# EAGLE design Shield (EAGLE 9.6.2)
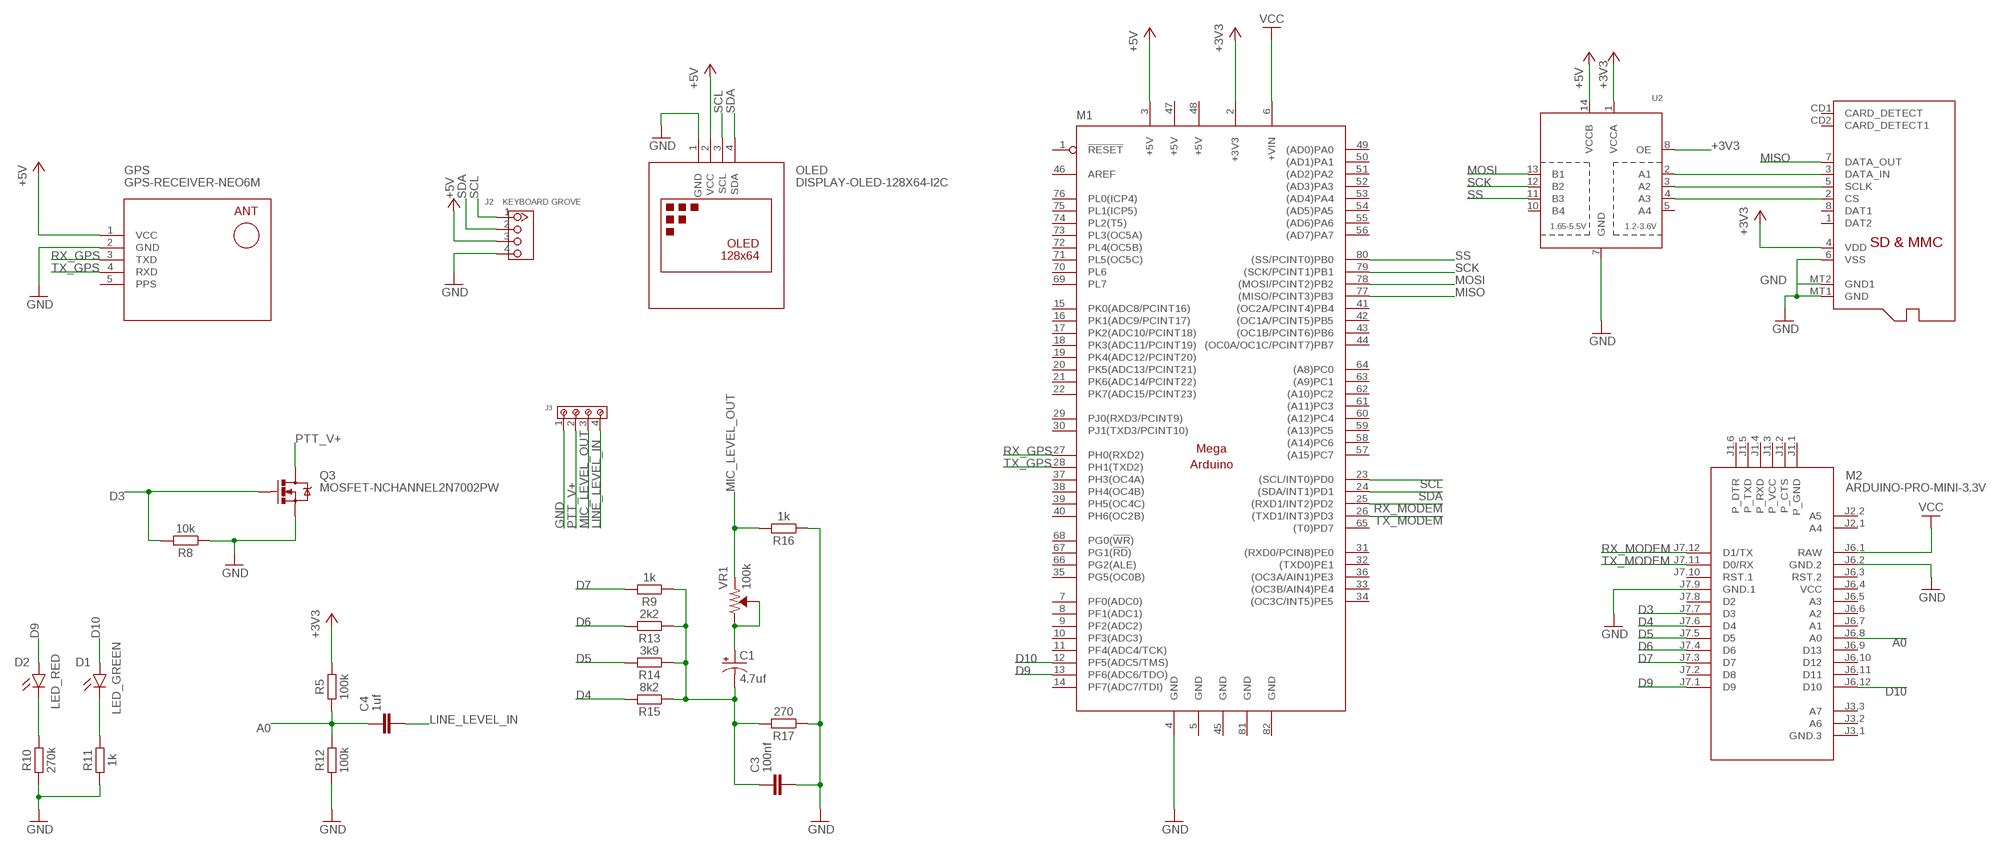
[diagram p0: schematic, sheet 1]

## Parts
C1  4.7uf  CPOL-USCT3528  [CT3528]
C3  100nf  C_CHIP-0805(2012-METRIC)  [CAPC2012X110]
C4  1uf  C_CHIP-0805(2012-METRIC)  [CAPC2012X110]
D1  LED_GREEN  CHIP-ROUND-R_0805  [LEDC2012X105N_RND-R]
D2  LED_RED  CHIP-ROUND-R_0805  [LEDC2012X105N_RND-R]
GPS  GPS-RECEIVER-NEO6M  [GPS-RECEIVER-NEO6M]
J2  KEYBOARD GROVE  GROVE-CONNECTOR-DIP-90D(4P-2.0)  [HW4-2.0-90D]
J3  691210910004  [691210910004]
M1  MEGAARDUINO_1  [MEGA_ARDUINO]
M2  ARDUINO-PRO-MINI-3.3V  [ARDUINO-PRO-MINI]
OLED  DISPLAY-OLED-128X64-I2C  [DISPLAY-OLED-128X64-I2C]
Q3  MOSFET-NCHANNEL2N7002PW  [SOT323]
R5  100k  R_CHIP-0805(2012-METRIC)  [RESC2012X65]
R8  10k  R_CHIP-0805(2012-METRIC)  [RESC2012X65]
R9  1k  R_CHIP-0805(2012-METRIC)  [RESC2012X65]
R10  270k  R_CHIP-0805(2012-METRIC)  [RESC2012X65]
R11  1k  R_CHIP-0805(2012-METRIC)  [RESC2012X65]
R12  100k  R_CHIP-0805(2012-METRIC)  [RESC2012X65]
R13  2k2  R_CHIP-0805(2012-METRIC)  [RESC2012X65]
R14  3k9  R_CHIP-0805(2012-METRIC)  [RESC2012X65]
R15  8k2  R_CHIP-0805(2012-METRIC)  [RESC2012X65]
R16  1k  R_CHIP-0805(2012-METRIC)  [RESC2012X65]
R17  270  R_CHIP-0805(2012-METRIC)  [RESC2012X65]
SD  MICROSD  [MICROSD]
U2  TXB0104PWR  [TSSOP14]
VR1  100k  TRIMPOT-SMD-3MM-CLOSED-1/8W-20%  [TRIMPOT-SMD-3MM-CLOSED]

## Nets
+3V3: M1.2(+3V3) R5.2 SD.4(VDD) U2.1(VCCA) U2.8(OE)
+5V: GPS.1(VCC) J2.3 M1.3(+5V) OLED.2(VCC) U2.14(VCCB)
A0: C4.1 M2.J6.8(A0) R5.1 R12.2
D3: M2.J7.7(D3) Q3.1(G) R8.2
D4: M2.J7.6(D4) R15.2
D5: M2.J7.5(D5) R14.2
D6: M2.J7.4(D6) R13.2
D7: M2.J7.3(D7) R9.2
D9: D2.A M1.13(PF6(ADC6/TDO)) M2.J7.1(D9)
D10: D1.A M1.12(PF5(ADC5/TMS)) M2.J6.12(D10)
GND: C3.2 GPS.2(GND) J2.4 J3.1 M1.4(GND) M2.J6.2(GND.2) M2.J7.9(GND.1) OLED.1(GND) Q3.2(S) R8.1 R10.1 R11.1 R12.1 R16.1 R17.1 SD.6(VSS) SD.MT1(GND) SD.MT2(GND1) U2.7(GND)
LINE_LEVEL_IN: C4.2 J3.4
LINE_LEVEL_OUT: C1.+ VR1.2(WIPER) VR1.3(CW)
MIC_LEVEL_OUT: J3.3 R16.2 VR1.1(CCW)
MISO: M1.77((MISO/PCINT3)PB3) SD.7(DATA_OUT)
MOSI: M1.78((MOSI/PCINT2)PB2) U2.13(B1)
N$1: SD.3(DATA_IN) U2.2(A1)
N$2: C1.- C3.1 R9.1 R13.1 R14.1 R15.1 R17.2
N$3: D2.C R10.2
N$4: D1.C R11.2
N$5: SD.5(SCLK) U2.3(A2)
N$6: SD.2(CS) U2.4(A3)
PTT_V+: J3.2 Q3.3(D)
RX_GPS: GPS.3(TXD) M1.27(PH0(RXD2))
RX_MODEM: M1.25((RXD1/INT2)PD2) M2.J7.12(D1/TX)
SCK: M1.79((SCK/PCINT1)PB1) U2.12(B2)
SCL: J2.1 M1.23((SCL/INT0)PD0) OLED.3(SCL)
SDA: J2.2 M1.24((SDA/INT1)PD1) OLED.4(SDA)
SS: M1.80((SS/PCINT0)PB0) U2.11(B3)
TX_GPS: GPS.4(RXD) M1.28(PH1(TXD2))
TX_MODEM: M1.26((TXD1/INT3)PD3) M2.J7.11(D0/RX)
VCC: M1.6(+VIN) M2.J6.1(RAW)
Unconnected: M1.1(!RESET) M1.7(PF0(ADC0)) M1.8(PF1(ADC1)) M1.9(PF2(ADC2)) M1.10(PF3(ADC3)) M1.11(PF4(ADC4/TCK)) M1.14(PF7(ADC7/TDI)) M1.15(PK0(ADC8/PCINT16)) M1.16(PK1(ADC9/PCINT17)) M1.17(PK2(ADC10/PCINT18)) M1.18(PK3(ADC11/PCINT19)) M1.19(PK4(ADC12/PCINT20)) M1.20(PK5(ADC13/PCINT21)) M1.21(PK6(ADC14/PCINT22)) M1.22(PK7(ADC15/PCINT23)) M1.29(PJ0(RXD3/PCINT9)) M1.30(PJ1(TXD3/PCINT10)) M1.31((RXD0/PCIN8)PE0) M1.32((TXD0)PE1) M1.33((OC3B/AIN4)PE4) M1.34((OC3C/INT5)PE5) M1.35(PG5(OC0B)) M1.36((OC3A/AIN1)PE3) M1.37(PH3(OC4A)) M1.38(PH4(OC4B)) M1.39(PH5(OC4C)) M1.40(PH6(OC2B)) M1.41((OC2A/PCINT4)PB4) M1.42((OC1A/PCINT5)PB5) M1.43((OC1B/PCINT6)PB6) M1.44((OC0A/OC1C/PCINT7)PB7) M1.46(AREF) M1.49((AD0)PA0) M1.50((AD1)PA1) M1.51((AD2)PA2) M1.52((AD3)PA3) M1.53((AD4)PA4) M1.54((AD5)PA5) M1.55((AD6)PA6) M1.56((AD7)PA7) M1.57((A15)PC7) M1.58((A14)PC6) M1.59((A13)PC5) M1.60((A12)PC4) M1.61((A11)PC3) M1.62((A10)PC2) M1.63((A9)PC1) M1.64((A8)PC0) M1.65((T0)PD7) M1.66(PG2(ALE)) M1.67(PG1(!RD!)) M1.68(PG0(!WR!)) M1.69(PL7) M1.70(PL6) M1.71(PL5(OC5C)) M1.72(PL4(OC5B)) M1.73(PL3(OC5A)) M1.74(PL2(T5)) M1.75(PL1(ICP5)) M1.76(PL0(ICP4)) M2.J1.1(P_GND) M2.J1.2(P_CTS) M2.J1.3(P_VCC) M2.J1.4(P_RXD) M2.J1.5(P_TXD) M2.J1.6(P_DTR) M2.J2.1(A4) M2.J2.2(A5) M2.J3.1(GND.3) M2.J3.2(A6) M2.J3.3(A7) M2.J6.3(RST.2) M2.J6.5(A3) M2.J6.6(A2) M2.J6.7(A1) M2.J6.9(D13) M2.J6.10(D12) M2.J6.11(D11) M2.J7.2(D8) M2.J7.8(D2) M2.J7.10(RST.1) SD.1(DAT2) SD.8(DAT1) SD.CD1(CARD_DETECT) SD.CD2(CARD_DETECT1) U2.5(A4) U2.10(B4)

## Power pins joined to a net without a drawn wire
+5V: M1.47(+5V) M1.48(+5V)
GND: M1.5(GND) M1.45(GND) M1.81(GND) M1.82(GND)
PPS: GPS.5(PPS)
VCC: M2.J6.4(VCC)

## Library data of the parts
C1 = adafruit:CPOL-US: POLARIZED CAPACITOR, American symbol
C3 C4 = Capacitor:C: Capacitor - Generic; CATEGORY: Capacitor
D1 = LED:CHIP-ROUND-R: LED - Generic; CATEGORY: LED; COLOR: RED; DESCRIPTION: CHIP LED ROUND; SUB-CATEGORY: CHIP; TYPE: ROUND_TOP; VALUE: LED_RED
D2 = LED:CHIP-ROUND-R: LED - Generic; CATEGORY: LED; COLOR: RED; DESCRIPTION: CHIP LED ROUND; SUB-CATEGORY: CHIP; TYPE: ROUND_TOP
GPS = diy-modules:GPS-RECEIVER-NEO6M: GPS Receiver Module based on NEO-6 device Short tutorial how to use NEO-6 module with Arduino: http://www.xarg.org/2016/06/neo6mv2-gps-module-with-arduino/ NEO-6 datasheet is available here: https://www.u-blox.com/sites/default/files/products/documents/NEO-6_DataSheet_%28GPS.G6-HW-09005%29.pdf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
J2 = OPL_Connector:GROVE-CONNECTOR-DIP-90D(4P-2.0): 320110034; VALUE: 4P-2.0-90D
J3 = Wurth_Connectors_WR-TBL Rising Cage Clamp:691210910004: WR-TBL Serie 2109 - 2.54 mm Horiz. Entry KIND PROPERTIES Pitch 2.54 mm MATERIAL PROPERTIES Insulator Material PA66 Insulator Flammability Rating UL94 V-0 Insulator Color Green Contact Material Brass Contact Plating Copper over Zinc Terminal Screw Material Steel Terminal Screw Plating Zinc Wire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; DATASHEET-URL: https://www.we-online.com/catalog/datasheet/691210910004.pdf; IR-UL: 6A; MOUNT: THT; PART-NUMBER: 691210910004; PINS: 4; PITCH: 2.54mm; TYPE: Horizontal; WIRE: 30 to 18 (AWG) 0.0509 to 0.823 (mm²); WORKING-VOLTAGE-UL: 150V (AC)
M1 = arduino:MEGAARDUINO_1: The Arduino Mega is a microcontroller board based on the ATmega1280. - 54 digital input/output pins (of which 14 can be used as PWM outputs) - 16 analog inputs - 4 UARTs (hardware serial ports) - 16 MHz crystal oscillator - USB connection - power jack - ICSP header - reset button It contains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
M2 = diy-modules:ARDUINO-PRO-MINI-*: Arduino Pro Mini and compatible devices More details available here: https://www.arduino.cc/en/Main/ArduinoBoardProMini Click here to find device on ebay.com
OLED = diy-modules:DISPLAY-OLED-128X64-I2C: 128x64 Dot Matrix OLED Module based on SSD1306 chip Variant with I2C interface More details available here: http://www.instructables.com/id/Monochrome-096-i2c-OLED-display-with-arduino-SSD13/ SSD1306 datasheet: https://cdn-shop.adafruit.com/datasheets/SSD1306.pdf Click here to find device on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
Q3 = BeagleBone_Blue_R3:MOSFET-NCHANNEL: Common NMOSFET Parts MFG P/NStore IDProd ID FDD8780TRANS-09984 SI7820DNTRANS-11055 FDS6630AIC-08089 2N7002PWTRANS-11151 FQP30N06L COM-10213TRANS-10060 BSS123LT1GTRANS-08345 BSS138TRANS-00830 BS170 2N7000; PROD_ID: TRANS-11151
R5 R8-R17 = Resistor:R: Resistor Fixed - Generic; CATEGORY: Resistor; SUB-CATEGORY: Fixed
SD = adafruit:MICROSD: Micro-SD / Transflash card holder with SPI pinout For the 3M # 2908-05WB-MG and/or 4UCON #19656 push-push type
U2 = adafruit:TXB0104PWR: 4-Bit Bi-Directional Level Shifter 1.2V-3.6V (VCCA) to 1.65V-5.5V (VCCB) bi-directional level shifter with auto direction sensing. Max data rate - VCCA 1.8V: 20Mbps (50ns), VCCA 3.3V: 100Mbps (10ns) Digikey: 296-21929-1-ND
VR1 = SparkFun-Resistors:TRIMPOT: Trimming Potentiometer (Trimpot) Three-terminal potentiometers, with an adjustable wiper and two adjustable resistors. A pot can be used to create a configurable voltage divider, or as a variable resistor. "Trimpots" are a subset of potentiometers, usually intended for "set-and-forget"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; PROD_ID: RES-09285; VALUE: 10k

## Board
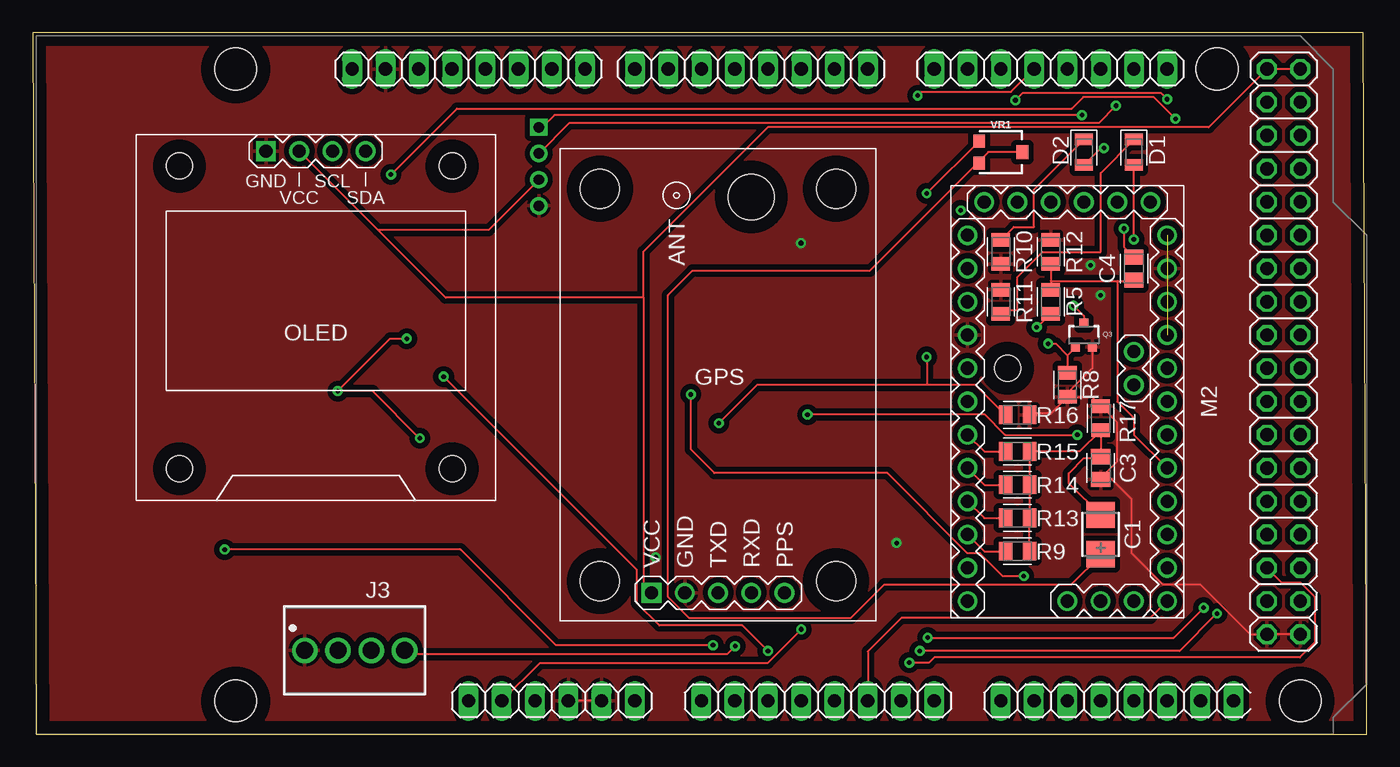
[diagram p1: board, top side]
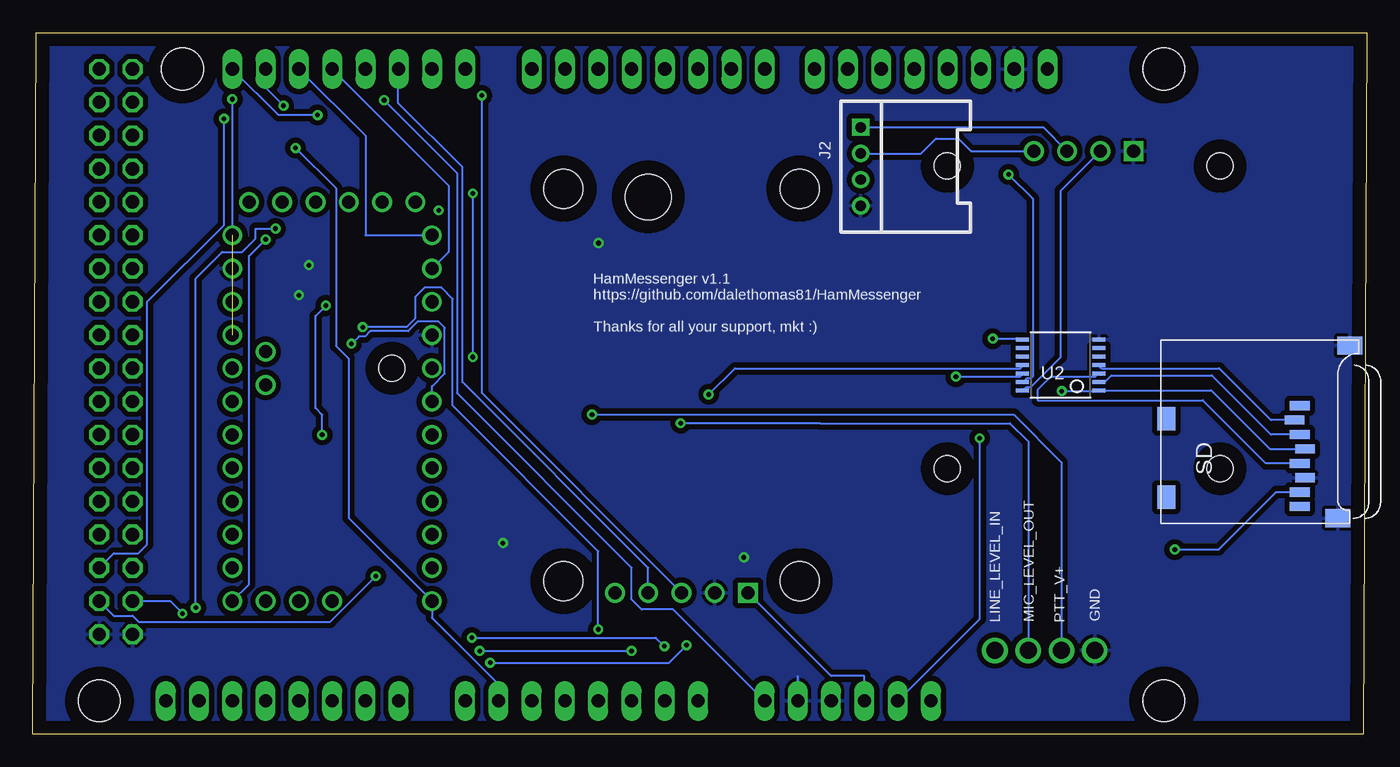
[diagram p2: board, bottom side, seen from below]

Size 101.85 x 53.57 mm. Coordinates in mm from the lower left corner, seen from the top.
Outline: 0.25,0 101.85,0 101.6,53.57 0,53.57 0.25,0
Copper layers (1*16): Top 0.035mm / dielectric 1.5mm / Bottom 0.035mm
Design rules "default": minimum track width 6mil, minimum drill 0.35mm, track to track 6mil, track to pad 6mil, pad to pad 6mil, via to via 6mil, smd to smd 6mil, copper to edge 40mil, drill to drill 6mil, minimum pad ring 10mil, minimum via ring 8mil, stop-mask expansion 4mil, vias tented up to drill 0mil, thermal gap 10mil

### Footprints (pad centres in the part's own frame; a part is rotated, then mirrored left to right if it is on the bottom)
CT3528 = smd 2 x 2.2: + 1.5,0; - -1.5,0
CAPC2012X110 = smd 1.165 x 1.465: 1 -0.875,0; 2 0.875,0
LEDC2012X105N_RND-R = smd 0.862 x 1.362: A 0.975,0; C -0.975,0
GPS-RECEIVER-NEO6M = drill 1 square: 1 -15.875,5.08 | drill 1: 2 -15.875,2.54; 3 -15.875,0; 4 -15.875,-2.54; 5 -15.875,-5.08 | hole 3: -14.986,9.017; -14.986,-9.017; 14.986,-9.017; 14.986,9.017 | hole 3.5: 14.351,-2.54
HW4-2.0-90D = drill 0.8 pad 1.27 square: 1 -3,0 | drill 0.8 pad 1.27: 2 -1,0; 3 1,0; 4 3,0
691210910004 = drill 1.3: 1 -3.81,0; 2 -1.27,0; 3 1.27,0; 4 3.81,0
MEGA_ARDUINO = drill 1.016 long: 1 33.02,2.54; 2 35.56,2.54; 3 38.1,2.54; 4 40.64,2.54; 5 43.18,2.54; 6 45.72,2.54; 7 50.8,2.54; 8 53.34,2.54; 9 55.88,2.54; 10 58.42,2.54; 11 60.96,2.54; 12 63.5,2.54; 13 66.04,2.54; 14 68.58,2.54; 15 73.66,2.54; 16 76.2,2.54; 17 78.74,2.54; 18 81.28,2.54; 19 83.82,2.54; 20 86.36,2.54; 21 88.9,2.54; 22 91.44,2.54; 23 86.36,50.8; 24 83.82,50.8; 25 81.28,50.8; 26 78.74,50.8; 27 76.2,50.8; 28 73.66,50.8; 29 71.12,50.8; 30 68.58,50.8; 31 63.5,50.8; 32 60.96,50.8; 33 58.42,50.8; 34 55.88,50.8; 35 53.34,50.8; 36 50.8,50.8; 37 48.26,50.8; 38 45.72,50.8; 39 41.91,50.8; 40 39.37,50.8; 41 36.83,50.8; 42 34.29,50.8; 43 31.75,50.8; 44 29.21,50.8; 45 26.67,50.8; 46 24.13,50.8 | drill 1.016 octagon: 47 93.98,50.8; 48 96.52,50.8; 49 93.98,48.26; 50 96.52,48.26; 51 93.98,45.72; 52 96.52,45.72; 53 93.98,43.18; 54 96.52,43.18; 55 93.98,40.64; 56 96.52,40.64; 57 93.98,38.1; 58 96.52,38.1; 59 93.98,35.56; 60 96.52,35.56; 61 93.98,33.02; 62 96.52,33.02; 63 93.98,30.48; 64 96.52,30.48; 65 93.98,27.94; 66 96.52,27.94; 67 93.98,25.4; 68 96.52,25.4; 69 93.98,22.86; 70 96.52,22.86; 71 93.98,20.32; 72 96.52,20.32; 73 93.98,17.78; 74 96.52,17.78; 75 93.98,15.24; 76 96.52,15.24; 77 93.98,12.7; 78 96.52,12.7; 79 93.98,10.16; 80 96.52,10.16; 81 93.98,7.62; 82 96.52,7.62 | hole 3.2: 15.24,50.8; 15.24,2.54; 90.17,50.8; 96.52,2.54 | hole 2: 74.168,27.94
ARDUINO-PRO-MINI = drill 1: J1.1 -15.24,6.35; J1.2 -15.24,3.81; J1.3 -15.24,1.27; J1.4 -15.24,-1.27; J1.5 -15.24,-3.81; J1.6 -15.24,-6.35; J2.1 -1.27,5.08; J2.2 -3.81,5.08; J3.1 15.24,0; J3.2 15.24,2.54; J3.3 15.24,5.08; J6.1 -12.7,7.62; J6.2 -10.16,7.62; J6.3 -7.62,7.62; J6.4 -5.08,7.62; J6.5 -2.54,7.62; J6.6 0,7.62; J6.7 2.54,7.62; J6.8 5.08,7.62; J6.9 7.62,7.62; J6.10 10.16,7.62; J6.11 12.7,7.62; J6.12 15.24,7.62; J7.1 15.24,-7.62; J7.2 12.7,-7.62; J7.3 10.16,-7.62; J7.4 7.62,-7.62; J7.5 5.08,-7.62; J7.6 2.54,-7.62; J7.7 0,-7.62; J7.8 -2.54,-7.62; J7.9 -5.08,-7.62; J7.10 -7.62,-7.62; J7.11 -10.16,-7.62; J7.12 -12.7,-7.62
DISPLAY-OLED-128X64-I2C = drill 1 square: 1 -3.81,12.7 | drill 1: 2 -1.27,12.7; 3 1.27,12.7; 4 3.81,12.7 | hole 2: -10.414,11.557; 10.414,11.557; 10.414,-11.557; -10.414,-11.557
SOT323 = smd 0.7 x 0.7: 1 -0.65,-0.925; 2 0.65,-0.925; 3 0,0.925
RESC2012X65 = smd 1.031 x 1.42: 1 -0.919,0; 2 0.919,0
MICROSD = smd 0.7 x 1.5: 1 9,-10.64; 2 7.9,-10.24; 3 6.8,-10.64; 4 5.7,-11.04; 5 4.6,-10.64; 6 3.5,-11.04; 7 2.4,-10.64; 8 1.3,-10.64 | smd 1.8 x 1.4: CD1 2,-0.44; CD2 8,-0.44 | smd 1.4 x 1.9: MT1 0.4,-13.54; MT2 13.6,-14.44
TSSOP14 = smd 0.305 x 0.991: 1 -1.95,-2.918; 2 -1.3,-2.918; 3 -0.65,-2.918; 4 0,-2.918; 5 0.65,-2.918; 6 1.3,-2.918; 7 1.95,-2.918; 8 1.95,2.918; 9 1.3,2.918; 10 0.65,2.918; 11 0,2.918; 12 -0.65,2.918; 13 -1.3,2.918; 14 -1.95,2.918
TRIMPOT-SMD-3MM-CLOSED = smd 1 x 0.9: 1 -0.85,-1.65; 3 0.85,-1.65 | smd 1.1 x 0.9: 2 0,1.65

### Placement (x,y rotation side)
C1  81.53,15.24 270 top
C3  81.53,20.32 270 top
C4  84.07,35.56 90 top
D1  84.07,44.45 270 top
D2  80.26,44.45 270 top
GPS  52.32,26.67 90 top
J2  38.64,43.35 270 bottom
J3  24.58,6.39 0 top
M1  0.25,0 0 top
M2  78.99,25.4 270 top
OLED  21.61,31.83 0 top
Q3  80.26,30.48 0 top
R5  77.72,33.02 270 top
R8  78.99,26.67 90 top
R9  75.18,13.97 180 top
R10  73.91,36.83 90 top
R11  73.91,33.02 270 top
R12  77.72,36.83 270 top
R13  75.18,16.51 180 top
R14  75.18,19.05 180 top
R15  75.18,21.59 180 top
R16  75.18,24.38 180 top
R17  81.53,24.13 270 top
SD  15.75,16.08 90 bottom
U2  23.37,28.19 90 bottom
VR1  73.91,44.45 270 top

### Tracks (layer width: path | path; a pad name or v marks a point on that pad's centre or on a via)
+3V3  (via drill 0.35)
  Top 0.152: v58.67,8 56.12,5.45 38.72,5.45 M1.2 | v76.65,31.08 76.7,31.08 R5.2 | v28.55,30.2 27.29,30.2 v23.29,26.19 25.96,26.19 v29.55,22.6
  Bottom 0.152: v58.67,8 58.67,13.97 69.79,25.08 69.79,33.23 70.65,34.1 71.95,34.1 72.65,33.4 72.65,31.76 72.64,31.75 73.31,31.08 v76.65,31.08 | v23.29,26.19 20.57,26.19 U2.1 20.43,26.26 11.89,26.26 7.41,21.78 SD.4 | v28.55,30.2 26.34,30.2 U2.8 | M1.2 29.55,8.8 v29.55,22.6
+5V
  Top 0.152: M1.48 M1.47 89.79,46.35 56.13,46.35 46.64,36.87 46.64,33.34 | GPS.1 46.64,11.39 46.64,33.34 | 26.36,38.51 31.54,33.34 46.64,33.34 | 26.36,38.51 OLED.2 | J2.3 34.8,38.51 26.36,38.51
  Bottom 0.152: GPS.1 40.89,4.45 38.35,4.45 M1.3 | U2.14 26.13,26.35 25.97,26.51 25.65,26.51 23.37,28.8 23.37,41.51 OLED.2
A0
  Top 0.152: R12.2 77.72,34.61 | 77.72,34.61 R5.1 | 77.72,34.61 82.8,34.61 | 82.8,34.61 84.07,34.61 C4.1 | M2.J6.8 84.07,22.86 84.07,24.13 82.8,25.4 82.8,34.61
D3  (via drill 0.35)
  Top 0.152: Q3.1 78.99,28.93 | 78.99,28.93 R8.2 | v77.52,29.83 78.1,29.83 78.99,28.93
  Bottom 0.152: M2.J7.7 71.37,26.55 70.39,27.53 70.39,31.04 70.85,31.5 72.46,31.5 73.19,30.77 76.08,30.77 76.48,30.38 76.95,30.38 77.49,29.83 v77.52,29.83
D4
  Top 0.152: M2.J7.6 72.64,21.59 R15.2
D5
  Top 0.152: M2.J7.5 72.64,19.05 R14.2
D6
  Top 0.152: M2.J7.4 72.64,16.51 R13.2
D7
  Top 0.152: M2.J7.3 72.64,13.97 R9.2
D9  (via drill 0.35)
  Top 0.152: v81.79,44.77 81.56,44.77 D2.A
  Bottom 0.152: M1.13 66.29,3.81 71.37,8.89 M2.J7.1 77.72,16.51 77.72,28.67 78.71,29.65 78.71,41.69 v81.79,44.77
D10  (via drill 0.35)
  Top 0.152: v84.07,37.78 D1.A | M1.12 63.75,6.32 66.33,8.89 85.34,8.89 M2.J6.12
  Bottom 0.152: v84.07,37.78 85.34,36.51 85.34,11.43 M2.J6.12
GND  (via drill 0.35)
  Top 0.152: M1.5 M1.4 | M1.82 M1.81 92.96,7.62 89.15,11.43 86.3,11.43 83.92,13.81 83.92,17.94 82.18,19.67 81.53,19.67 | 81.53,25.08 R17.1 | R8.1 78.99,26.04 80.91,27.96 Q3.2 | R16.1 76.2,24.48 77.72,24.48 R8.1 | C3.2 81.53,19.56 82.8,20.83 82.8,23.81 81.53,25.08 | R8.1 80.87,25.75 81.53,25.08
  Bottom 0.152: M1.5 43.43,4.45
  other vias: 80.77,35.81 81.53,33.53 58.65,37.5 47.55,13.5 65.95,14.6
  pour Top (isolate 0.406): 0.25,53.34 0.25,0 101.85,0 101.85,53.34
  pour Bottom (isolate 0.406): 0.25,53.59 101.85,53.59 101.85,0 0.25,0
LINE_LEVEL_IN  (via drill 0.35)
  Top 0.152: v53.63,6.71 53.02,6.1 28.69,6.1 J3.4 | v68.33,7.37 87.12,7.37 v89.41,9.65 | v83.31,38.61 83.31,37.2 C4.2
  Bottom 0.152: v89.41,9.65 89.41,34.8 87.38,36.83 85.85,36.83 84.84,37.85 84.84,38.61 v83.31,38.61 | v53.63,6.71 54.29,7.37 v68.33,7.37
LINE_LEVEL_OUT
  Top 0.152: VR1.2 72.96,44.45 72.33,43.81 VR1.3 72.01,43.5 63.91,35.4 50.39,35.4 48.51,33.53 48.51,10.48 50.1,8.89 62.48,8.89 65.02,11.43 79.31,11.43 81.53,13.65 C1.+
MIC_LEVEL_OUT  (via drill 0.35)
  Top 0.152: R16.2 71.98,26.67 68.25,26.67 | v52.39,23.75 55.31,26.67 68.25,26.67 | VR1.1 v68.26,41.3 v68.25,41.3 | v68.25,28.8 68.25,26.67
  Bottom 0.152: J3.3 25.85,22.36 27.23,23.74 41.73,23.74 41.73,23.75 v52.39,23.75 | v68.25,41.3 v68.25,28.8
MISO  (via drill 0.35)
  Top 0.152: v66.93,5.46 68.43,5.46 68.83,5.86 96.74,5.86 97.89,7 97.89,10.48 96.77,11.59 95.34,11.59 M1.77 | v51.94,6.79 39.96,6.79 32.65,14.1 v14.65,14.1
  Bottom 0.152: SD.7 6.91,18.48 11.29,14.1 v14.65,14.1 | v51.94,6.79 53.27,5.46 v66.93,5.46
MOSI  (via drill 0.35)
  Top 0.152: v87.25,46.99 85.58,48.66 80.2,48.66 79.33,47.78 32.38,47.78 v27.35,42.74
  Bottom 0.152: v27.35,42.74 25.5,40.89 25.5,27.3 25.65,27.15 25.97,27.15 26.13,26.99 U2.13 | v87.25,46.99 87.25,38.89 93.12,33.02 93.12,14.48 93.79,13.81 95.66,13.81 M1.78
N$1
  Bottom 0.152: U2.2 20,26.89 19.5,27.4 11.83,27.4 7.31,22.88 SD.3
N$2
  Top 0.152: R9.1 R13.1 R14.1 R15.1 79.91,21.59 R17.2 C3.1 81.53,21.08 80.26,21.08 79.11,19.93 79.11,19.16 C1.-
N$3
  Top 0.152: D2.C 80.26,45.4 76.45,41.59 76.45,38.73 74.9,38.73 R10.2
N$4
  Top 0.152: D1.C 84.07,45.4 81.53,42.86 81.53,36.83 77.09,36.83 75.18,34.92 75.18,32.38 73.91,32.38 R11.2
N$5
  Bottom 0.152: SD.5 7.71,20.68 12.51,25.48 25.12,25.48 25.12,26.31 24.13,27.3 20.73,27.3 20.57,27.46 U2.3
N$6
  Bottom 0.152: SD.2 7.31,23.98 11.27,27.94 20.26,27.94 20.42,28.1 U2.4
N$7  (via drill 0.35)
  other vias: 70.85,40
PTT_V+  (via drill 0.35)
  Top 0.152: v79.76,22.86 74.24,22.86 72.68,24.42 59.17,24.42 v59.15,24.4 | v79.47,32.73 80.26,31.94 Q3.3
  Bottom 0.152: v79.76,22.86 79.76,24.38 80.26,24.89 80.26,31.94 v79.47,32.73 | v59.15,24.4 26.95,24.4 23.31,20.76 J3.2
RX_GPS  (via drill 0.35)
  Top 0.152: v67.56,48.77 67.84,49.05 74.7,49.05 M1.27
  Bottom 0.152: GPS.3 67.56,26.04 v67.56,48.77
RX_MODEM
  Bottom 0.152: M2.J7.12 76.45,38.1 76.45,45.72 M1.25
SCK  (via drill 0.35)
  Top 0.152: v31.37,27.3 46.13,12.54 46.13,10 47.84,8.3 54.19,8.3 v56.13,6.35 | v67.72,6.35 87.57,6.35 v90.42,9.21
  Bottom 0.152: v31.37,27.3 26.45,27.3 26.29,27.46 U2.12 | v67.72,6.35 v56.13,6.35 | v90.42,9.21 91.38,10.16 M1.79
SCL  (via drill 0.35)
  Top 0.152: v80.11,47.28 39.83,47.28 38.9,46.35 J2.1
  Bottom 0.152: v80.11,47.28 83.09,47.28 M1.23 | J2.1 24.7,46.35 OLED.3
SDA  (via drill 0.35)
  Top 0.152: v82.7,48 v82.7,47.99 81.39,46.67 40.97,46.67 J2.2
  Bottom 0.152: v82.7,48 84.07,49.37 M1.24 | J2.2 34.02,44.35 32.89,45.48 31.16,45.48 30.21,44.53 OLED.4
SS  (via drill 0.35)
  Top 0.152: v50.25,25.94 50.25,21.74 52.05,19.94 65.24,19.94 71.37,13.81 72.33,13.81 74.07,12.06 v75.66,12.06
  Bottom 0.152: v50.25,25.94 48.25,27.94 26.45,27.94 26.29,28.1 U2.11 | v75.66,12.06 79.15,8.57 93.76,8.57 94.23,9.05 95.66,9.05 M1.80
TX_GPS
  Bottom 0.152: GPS.4 54.86,12.7 69.05,26.89 69.05,43.3 73.95,48.2 73.95,50.76 M1.28
TX_MODEM
  Bottom 0.152: M2.J7.11 70.1,36.83 70.1,41.91 M1.26
VCC  (via drill 0.35)  (1 unrouted)
  Top 0.152: v75.03,48.42 75.57,48.97 86.15,48.97 86.15,48.95 v86.61,48.49
  Bottom 0.152: M1.6 52.96,9.53 55.37,9.53 56.13,10.29 56.13,12.7 69.47,26.04 69.47,42.86 v75.03,48.42 | v86.61,48.49 M2.J6.1

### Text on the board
bPlace: HamMessenger v1.1 / https://github.com/dalethomas81/HamMessenger / / Thanks for all your support, mkt :) | MIC_LEVEL_OUT | LINE_LEVEL_IN | PTT_V+ | GND

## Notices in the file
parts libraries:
diy-modules: Released under the Creative Commons Attribution 4.0 International License: http://creativecommons.org/licenses/by/4.0
SparkFun-Resistors: Licensing: Creative Commons ShareAlike 4.0 International - https://creativecommons.org/licenses/by-sa/4.0
